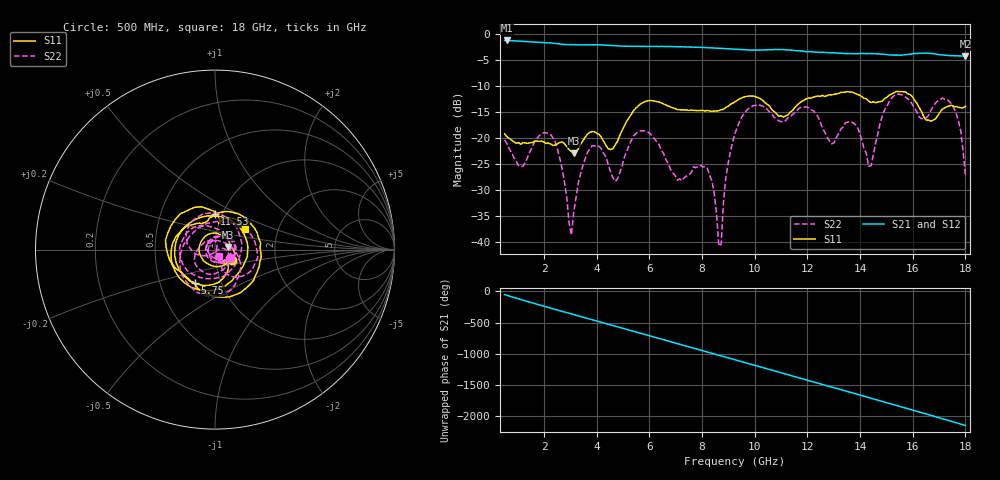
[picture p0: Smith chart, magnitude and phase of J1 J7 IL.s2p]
!Agilent Technologies,N5230A,MY45001360,A.07.50.67
!Agilent N5230A: A.07.50.67
!Date: Tuesday, April 16, 2024 17:45:52
!Correction: S11(Full 2 Port(1,2))
!S21(Full 2 Port(1,2))
!S12(Full 2 Port(1,2))
!S22(Full 2 Port(1,2))
!S2P File: Measurements: S11, S21, S12, S22:
# Hz S  dB  R 50
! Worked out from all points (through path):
!   201 points, 500 MHz to 18 GHz, reference 50 ohm
!   highest |S21| = -1.22 dB at 587.5 MHz (marker M1); lowest = -4.2 dB at 18 GHz (marker M2)
!   group delay of S21, straight-line fit = 331 ps
!   lowest |S11| = -23.0 dB at 3.125 GHz (marker M3), VSWR 1.15, Z = 57.5 + j1.71 ohm
!   |S11| at or under -10 dB: start of sweep to end of sweep
!   |S22| runs from -40.9 to -11.5 dB; largest |S21 - S12| = 0.008
!   S11 on the Smith chart (normalised r, x): 500 MHz: 1.20, -0.14; 5.75 GHz: 0.75, -0.30; 11.53 GHz: 0.92, +0.38; 18 GHz: 1.35, +0.32
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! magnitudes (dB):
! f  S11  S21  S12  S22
! 500 MHz  -19.2  -1.2  -1.2  -20.4
! 587.5 MHz  -19.8  -1.2  -1.2  -21.1
! 2.25 GHz  -21.2  -1.7  -1.7  -19.4
! 3.038 GHz  -22.7  -2.0  -2.0  -38.7
! 3.125 GHz  -23.0  -2.0  -2.0  -34.3
! 3.475 GHz  -20.6  -2.1  -2.1  -25.3
! 4.088 GHz  -19.3  -2.0  -2.1  -21.6
! 4.7 GHz  -21.4  -2.2  -2.2  -28.4
! 5.75 GHz  -13.2  -2.4  -2.4  -18.6
! 6.362 GHz  -13.1  -2.4  -2.4  -21.3
! 7.062 GHz  -14.6  -2.4  -2.4  -28.2
! 8.2 GHz  -14.7  -2.6  -2.6  -25.9
! 8.637 GHz  -14.8  -2.7  -2.7  -40.9
! 9.25 GHz  -13.0  -2.9  -2.9  -19.1
! 11.53 GHz  -14.1  -3.2  -3.1  -15.1
! 12.22 GHz  -12.2  -3.4  -3.4  -14.8
! 12.93 GHz  -11.7  -3.6  -3.6  -21.2
! 13.8 GHz  -11.4  -3.8  -3.8  -17.3
! 14.32 GHz  -12.9  -3.7  -3.7  -25.5
! 15.11 GHz  -11.7  -4.0  -4.0  -12.9
! 17.39 GHz  -13.8  -4.1  -4.2  -13.0
! 18 GHz  -13.9  -4.2  -4.3  -27.3
